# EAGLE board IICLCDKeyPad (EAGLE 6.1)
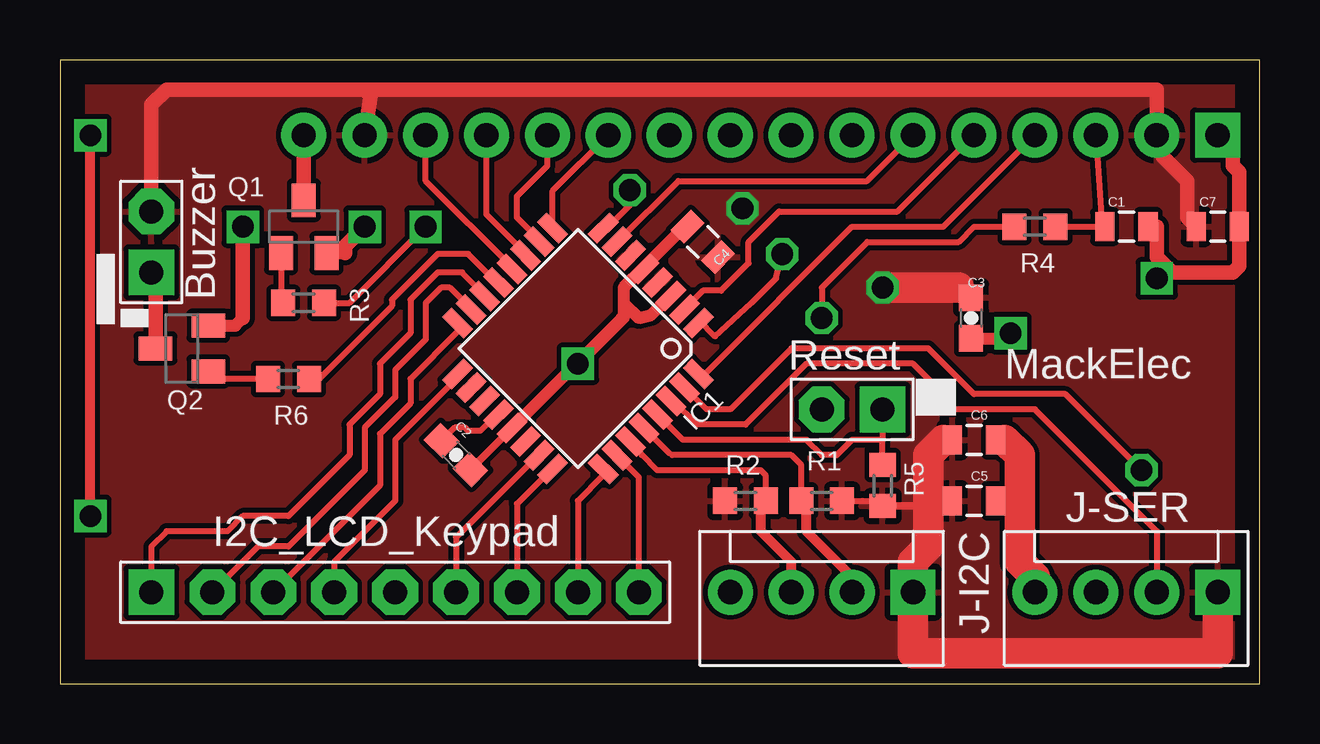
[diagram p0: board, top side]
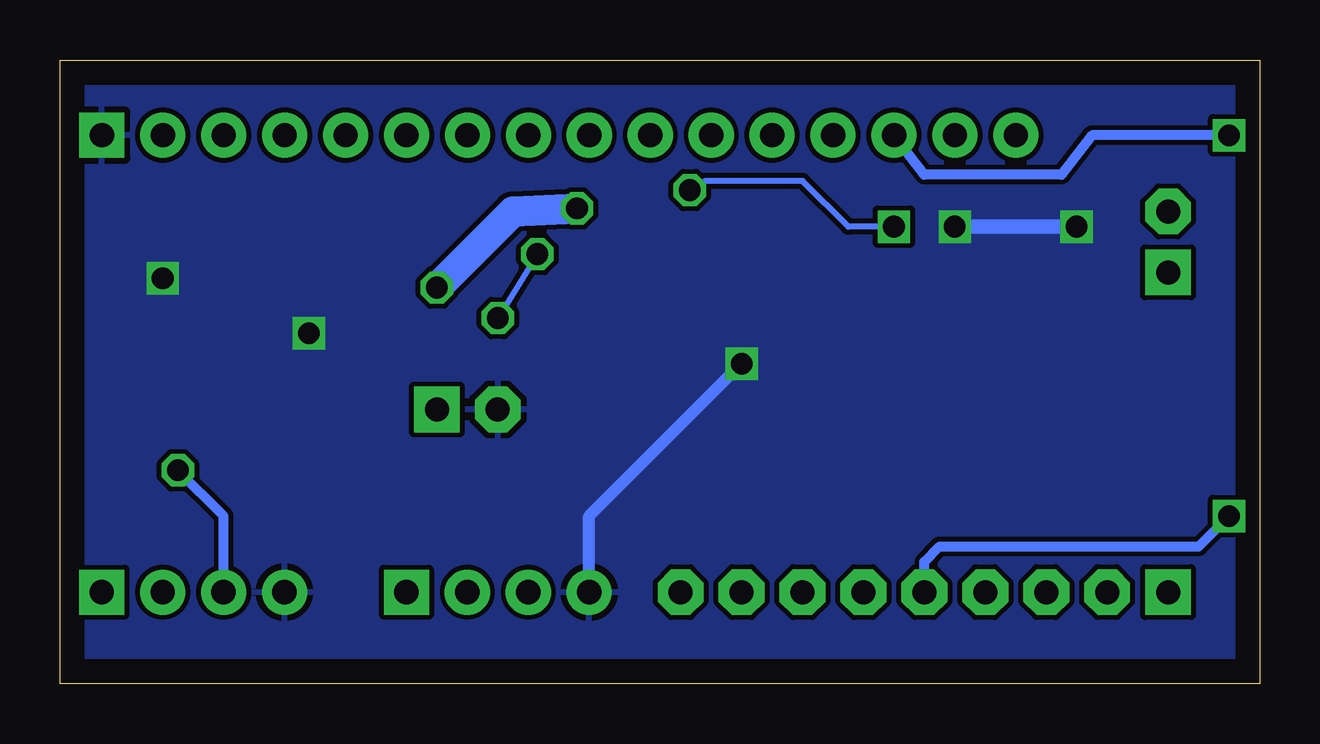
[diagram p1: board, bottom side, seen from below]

Size 50 x 26 mm. Coordinates in mm from the lower left corner, seen from the top.
Outline: 0,0 50,0 50,26 0,26 0,0
Copper layers (1*16): Top 0.035mm / dielectric 1.5mm / Bottom 0.035mm
Design rules: minimum track width 10mil, minimum drill 24mil, track to track 8mil, track to pad 8mil, pad to pad 8mil, via to via 8mil, smd to smd 8mil, copper to edge 40mil, drill to drill 8mil, minimum pad ring 10mil, minimum via ring 8mil, stop-mask expansion 4mil, vias tented up to drill 0mil, thermal gap 10mil

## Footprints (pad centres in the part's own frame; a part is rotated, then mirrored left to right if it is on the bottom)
0805 = smd 0.8 x 1.2: 1 -0.9,0; 2 0.9,0
0603-CAP = smd 1.1 x 1: 1 -0.85,0; 2 0.85,0
TQFP32-08 = smd 1.27 x 0.559: 1 -4.293,2.8; 2 -4.293,2; 3 -4.293,1.2; 4 -4.293,0.4; 5 -4.293,-0.4; 6 -4.293,-1.2; 7 -4.293,-2; 8 -4.293,-2.8; 17 4.293,-2.8; 18 4.293,-2; 19 4.293,-1.2; 20 4.293,-0.4; 21 4.293,0.4; 22 4.293,1.2; 23 4.293,2; 24 4.293,2.8 | smd 0.559 x 1.27: 9 -2.8,-4.293; 10 -2,-4.293; 11 -1.2,-4.293; 12 -0.4,-4.293; 13 0.4,-4.293; 14 1.2,-4.293; 15 2,-4.293; 16 2.8,-4.293; 25 2.8,4.293; 26 2,4.293; 27 1.2,4.293; 28 0.4,4.293; 29 -0.4,4.293; 30 -1.2,4.293; 31 -2,4.293; 32 -2.8,4.293
SIL-9 = drill 1 pad 1.905 square: 1 -11.43,0 | drill 1 pad 1.905 octagon: 2 -8.89,0; 3 -6.35,0; 4 -3.81,0; 5 -1.27,0; 6 1.27,0; 7 3.81,0; 8 6.35,0; 9 8.89,0
MOLEX-4 = drill 1.016 pad 1.88 square: 1 -3.81,0 | drill 1.016 pad 1.88: 2 -1.27,0; 3 1.27,0; 4 3.81,0
JP1 = drill 1 pad 1.905 square: 1 -1.27,0 | drill 1 pad 1.905 octagon: 2 1.27,0
SOT23-BEC = smd 1 x 1.4: B -0.95,-1.1; C 0,1.1; E 0.95,-1.1
R0603 = smd 1 x 1.1: 1 -0.85,0; 2 0.85,0
LCD-16X2_BARE = drill 1.016 pad 1.88 square: 1 0.004,0.006 | drill 1.016 pad 1.88: 2 2.544,0.006; 3 5.084,0.006; 4 7.624,0.006; 5 10.164,0.006; 6 12.704,0.006; 7 15.244,0.006; 8 17.784,0.006; 9 20.324,0.006; 10 22.864,0.006; 11 25.404,0.006; 12 27.944,0.006; 13 30.484,0.006; 14 33.024,0.006; 15 35.564,0.006; 16 38.104,0.006

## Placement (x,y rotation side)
C1  10u  [0805]  44.45,19.05 0 top
C2  [0603-CAP]  16.51,9.53 315 top
C3  [0603-CAP]  37.97,15.24 270 top
C4  10u  [0805]  26.8,18.41 135 top
C5  10u  [0805]  38.1,7.62 0 top
C6  10u  [0805]  38.1,10.16 0 top
C7  10u  [0805]  48.26,19.05 0 top
IC1  MEGA8-AI  [TQFP32-08]  21.59,13.97 225 top
J1  SIL-9  [SIL-9]  15.24,3.81 0 top
J-I2C  MO4POL  [MOLEX-4]  31.75,3.81 180 top
J-SER  MO4POL  [MOLEX-4]  44.45,3.81 180 top
JP1  JP1  [JP1]  3.81,18.41 90 top
JP2  JP1  [JP1]  33.02,11.43 180 top
Q1  8050  [SOT23-BEC]  10.16,19.05 0 top
Q2  8050  [SOT23-BEC]  5.08,13.97 90 top
R1  4k7  [R0603]  31.75,7.62 0 top
R2  4k7  [R0603]  28.57,7.62 180 top
R3  1k  [R0603]  10.16,15.88 180 top
R4  1k  [R0603]  40.64,19.05 0 top
R5  10k  [R0603]  34.29,8.26 90 top
R6  10k  [R0603]  9.53,12.7 0 top
U1  LCD-20X4BARE  [LCD-16X2_BARE]  48.26,22.86 0 bottom

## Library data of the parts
C1-C7 = SparkFun-Passives
IC1 = atmel; MPN: ATMEGA8-16AU; OC_FARNELL: 9171371; OC_NEWARK: 73M8863
J1 J-I2C J-SER JP1 JP2 = Andrew Connectors
Q1 Q2 = transistor-npn
R1-R6 = rcl
U1 = Andrew Misc

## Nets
BL: IC1.8 R3.1
BUZZER: IC1.13 R6.2
C2: IC1.23 J1.6
C3: IC1.24 J1.7
C4: IC1.25 J1.8
C5: IC1.26 J1.9
D6: IC1.11 U1.13
E: IC1.7 U1.6
GND: C1.2 C2.2 C3.2 C4.2 C5.2 C6.2 C7.2 IC1.3 IC1.5 IC1.21 J-I2C.4 J-SER.4 JP2.2 Q1.E Q2.E U1.1
N$1: IC1.14 J1.1
N$2: Q1.C U1.16
N$3: Q1.B R3.2
N$4: C1.1 R4.2 U1.3
N$5: IC1.9 U1.11
N$6: C2.1 IC1.20
N$7: IC1.10 U1.12
N$8: IC1.1 R4.1
N$9: IC1.32 U1.4
N$11: JP1.1 Q2.C
N$12: Q2.B R6.1
N$13: IC1.2 U1.5
N$14: IC1.15 J1.2
N$16: IC1.29 JP2.1 R5.2
N$17: IC1.16 J1.3
N$18: IC1.17 J1.4
N$20: IC1.12 J1.5 U1.14
RX: IC1.30 J-SER.2
SCL: IC1.28 J-I2C.2 R1.1
SDA: IC1.27 J-I2C.3 R2.1
TX: IC1.31 J-SER.3
VCC: C3.1 C4.1 C5.1 C6.1 C7.1 IC1.4 IC1.6 IC1.18 J-I2C.1 J-SER.1 JP1.2 R1.2 R2.2 R5.1 U1.2 U1.15

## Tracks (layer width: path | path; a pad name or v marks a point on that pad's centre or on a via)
BL  (via drill 0.9)
  Top 0.254: R3.1 12.06,15.88 v15.24,19.05 | v23.75,20.57 24.13,20.32 22.8,18.98 IC1.8
  Bottom 0.254: v15.24,19.05 17.14,19.05 19.05,20.95 23.11,20.95 v23.75,20.57
BUZZER
  Top 0.254: IC1.13 18.2,16.72 17.02,17.91 15.75,17.91 13.84,16 13.84,15.75 10.79,12.7 R6.2
C2
  Top 0.254: IC1.23 19.71,9.3 16.51,6.1 J1.6
C3
  Top 0.254: IC1.24 20.54,8.98 19.05,7.49 J1.7
C4
  Top 0.254: IC1.25 22.64,8.68 21.59,7.62 J1.8
C5
  Top 0.254: J1.9 24.13,8.6 IC1.26
D6
  Top 0.254: IC1.11 19.4,17.93 17.78,19.56 U1.13
E
  Top 0.254: U1.6 33.65,20.95 25.78,20.95 23.25,18.42 IC1.7
GND  (via drill 0.9)
  Top 0.254: C4.2 26.16,19.18
  Top 0.305: 39.37,10.16 C6.2 | C5.2 40.01,7.62 | C2.2 IC1.21
  Top 0.508: 23.5,15.88 23.5,16.51 24.27,17.29 IC1.5 24.34,17.36 26.16,19.18 | 23.5,15.88 24.13,15.24 24.64,15.37 25.35,16.08 IC1.3 | 23.5,15.88 23.5,15.24 | 23.5,15.24 23.43,15.24 IC1.21 | v21.59,13.34 23.5,15.24 | Q2.E 7.3,14.92 7.62,15.24 | Q1.E 11.89,17.95 | C3.2 39.41,14.39 v39.62,14.61
  Top 0.61: 11.89,17.95 11.89,18.25 v12.7,19.05 | v7.62,19.05 7.62,15.24 | U1.1 48.9,22.73 48.9,21.59 49.16,21.32 C7.2 49.16,17.41 48.9,17.14 46.35,17.14 45.72,17.78 45.72,19.05 C1.2
  Top 1.27: J-SER.4 40.64,4.45 40.01,5.08 40.01,7.62 40.01,9.53 39.37,10.16
  Bottom 0.508: J-I2C.4 27.94,6.99 v21.59,13.34
  Bottom 0.61: v12.7,19.05 v7.62,19.05
  other vias: 45.72,16.89
  pour Bottom: 0.64,25.4 49.53,25.4 49.53,0.64 0.64,0.64
N$1
  Top 0.254: IC1.14 17.75,16.16 16.76,17.14 15.75,17.14 14.61,16 14.61,14.61 13.34,13.34 13.34,12.06 12.06,10.79 12.06,9.53 9.53,6.99 7.62,6.99 6.99,6.35 4.45,6.35 3.81,5.71 J1.1
N$2
  Top 0.61: Q1.C U1.16
N$3
  Top 0.254: Q1.B 9.21,16.19 9.53,15.88 R3.2
N$4
  Top 0.254: R4.2 C1.1 43.43,19.17 U1.3
N$5
  Top 0.254: IC1.9 20.54,20.55 U1.11
N$6
  Top 0.254: IC1.20 18.2,11.22 17.53,10.54 17.02,10.54 16.89,10.67 16.45,10.67 C2.1
N$7
  Top 0.254: IC1.10 19.97,18.51 19.05,19.43 19.05,20.32 20.32,21.59 U1.12
N$8  (via drill 0.9)
  Top 0.254: IC1.1 26.61,15.18 27.3,14.48 28.83,15.88 29.84,16.89 v30.1,17.91 | R4.1 38.1,19.05 37.47,18.41 33.66,18.41 31.75,16.51 v31.75,15.24
  Bottom 0.254: v30.1,17.91 v31.75,15.24
N$9
  Top 0.254: IC1.32 26.89,12.91 33.02,19.05 36.82,19.05 U1.4
N$11
  Top 0.61: Q2.C 3.98,16.98 JP1.1
N$12
  Top 0.254: R6.1 6.5,12.7 Q2.B
N$13
  Top 0.254: IC1.2 26.29,15.88 26.8,16.38 27.56,16.38 28.7,17.53 28.7,18.41 29.97,19.68 34.91,19.68 U1.5
N$14
  Top 0.254: IC1.15 16.89,15.88 16.26,16.51 15.88,16.51 15.24,15.88 15.24,14.35 13.97,13.08 13.97,11.94 12.7,10.67 12.7,8.89 9.53,5.71 8.26,5.71 J1.2
N$16
  Top 0.254: R5.2 34.29,10.16 | JP2.1 34.29,10.16 | 34.29,10.16 33.02,10.16 32.38,9.53 31.75,9.53 31.11,10.16 25.97,10.16 IC1.29
N$17
  Top 0.254: IC1.16 16.57,14.67 14.61,12.7 14.61,11.68 13.34,10.41 13.34,8.26 J1.3
N$18
  Top 0.254: IC1.17 16.57,12.77 13.97,10.16 13.97,7.62 11.43,5.08 J1.4
N$20  (via drill 0.9)
  Top 0.254: IC1.12 18.84,17.36 15.24,20.95 U1.14
  Top 0.406: v1.27,6.99 v1.27,22.86
  Bottom 0.406: J1.5 13.97,5.08 13.34,5.71 2.54,5.71 v1.27,6.99 | v1.27,22.86 6.99,22.86 8.26,21.21 13.97,21.21 U1.14
RX
  Top 0.254: IC1.30 25.55,11.78 26.54,10.79 28.57,10.79 31.11,13.34 35.56,13.34 36.83,12.06 36.83,11.43 40.64,11.43 45.72,6.35 J-SER.2
SCL
  Top 0.254: R1.1 30.9,9.11 30.48,9.53 25.53,9.53 25.4,9.59 IC1.28
  Top 0.406: J-I2C.2 33.02,4.45 31.11,6.35 31.11,7.41 R1.1
SDA
  Top 0.254: R2.1 29.43,8.68 29.21,8.89 24.89,8.89 24.26,9.53 24.13,9.73 IC1.27
  Top 0.406: J-I2C.3 30.48,5.08 29.21,6.35 29.21,7.41 R2.1
TX  (via drill 0.9)
  Top 0.254: IC1.31 26.96,11.43 27.94,11.43 30.48,13.97 36.2,13.97 38.1,12.06 41.91,12.06 v45.09,8.89
  Bottom 0.406: J-SER.3 43.18,6.99 v45.09,8.89
VCC  (via drill 0.9)
  Top 0.254: R1.2 34.08,7.62 R5.1
  Top 0.305: C5.1 36.2,7.62 35.98,7.41 R5.1 | C6.1 36.83,10.16
  Top 0.406: IC1.6 23.9,17.93
  Top 0.61: JP1.2 3.81,24.13 4.45,24.77 12.7,24.77 | 12.7,24.77 45.72,24.77 45.72,23.37 U1.2 45.97,21.98 46.99,20.95 46.99,19.42 C7.1 | U1.15 12.95,24.52 12.7,24.77
  Top 1.27: 36.83,10.16 36.2,9.53 36.2,7.62 36.2,5.71 35.56,5.08 J-I2C.1 35.56,1.27 48.26,1.27 J-SER.1 | v34.29,16.51 37.47,16.51
  Bottom 1.27: v28.45,19.81 31.11,19.68 v34.29,16.51
  pour Top: 0.64,25.4 49.53,25.4 49.53,0.64 0.64,0.64

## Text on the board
tPlace: Buzzer | Reset | MackElec | I2C_LCD_Keypad

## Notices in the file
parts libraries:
SparkFun-Passives: Licensing: CC v3.0 Share-Alike You are welcome to use this library for commercial purposes.
